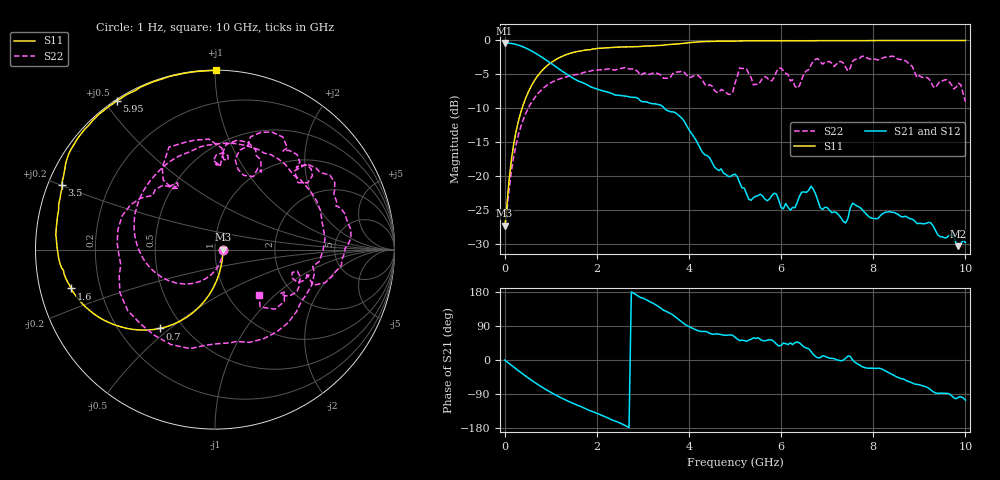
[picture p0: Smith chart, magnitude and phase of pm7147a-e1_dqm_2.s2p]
# GHz S DB R 50
! S-Parameters data
! Freq  dbS11  angS11  dbS21  angS21  dbS12  angS12  dbS22  angS22
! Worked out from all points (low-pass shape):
!   279 points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, 1 Hz to 10 GHz, reference 50 ohm
!   highest |S21| = -0.38 dB at 2 Hz (marker M1); lowest = -30.3 dB at 9.85 GHz (marker M2)
!   |S21| within 3 dB of the highest: start of sweep to 1.004 GHz
!   lowest |S11| = -27.3 dB at 1.6 Hz (marker M3), VSWR 1.09, Z = 54.5 - j1.04e-07 ohm
!   |S11| at or under -10 dB: start of sweep to 380.1 MHz
!   |S22| runs from -27.3 to -2.3 dB; largest |S21 - S12| = 0
!   S11 on the Smith chart (normalised r, x): 1 Hz: 1.09, -0.00; 700 MHz: 0.37, -0.46; 1.6 GHz: 0.09, -0.13; 3.5 GHz: 0.04, +0.20; 5.95 GHz: 0.00, +0.54; 10 GHz: 0.00, +1.01
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1e-09  -27.30 -0.0  -0.38 -0.0  -0.38 -0.0  -27.30 -0.0
1.6e-09  -27.30 -0.0  -0.38 -0.0  -0.38 -0.0  -27.30 -0.0
2e-09  -27.30 -0.0  -0.38 -0.0  -0.38 -0.0  -27.30 -0.0
0.25  -13.38 -92.7  -0.61 -23.6  -0.61 -23.6  -15.33 -108.1
0.7  -5.40 -125.1  -2.02 -62.9  -2.02 -62.9  -8.03 -170.7
1.6  -1.61 -164.9  -6.01 -120.1  -6.01 -120.1  -5.01 105.0
1.7  -1.49 -167.9  -6.25 -125.4  -6.25 -125.4  -4.75 98.0
2.65  -0.96 169.9  -8.24 -175.0  -8.24 -175.0  -4.06 20.4
3.35  -0.75 158.9  -9.48 140.2  -9.48 140.2  -4.95 -61.2
3.5  -0.66 157.1  -10.25 129.0  -10.25 129.0  -5.58 -80.7
3.9  -0.43 151.4  -11.95 95.3  -11.95 95.3  -4.70 -155.6
4.3  -0.20 145.0  -16.55 75.3  -16.55 75.3  -5.96 145.3
5.05  -0.10 134.4  -20.10 55.3  -20.10 55.3  -5.31 122.7
5.3  -0.06 131.1  -23.42 52.6  -23.42 52.6  -4.93 86.1
5.95  -0.06 123.5  -23.58 37.2  -23.58 37.2  -4.12 78.5
6.3  -0.05 119.7  -24.67 45.5  -24.67 45.5  -6.75 62.2
6.7  -0.06 115.9  -21.94 14.3  -21.94 14.3  -3.06 68.5
7.4  -0.04 109.2  -26.92 4.5  -26.92 4.5  -3.92 35.8
8.35  -0.03 101.3  -25.24 -34.4  -25.24 -34.4  -2.42 11.0
8.85  -0.02 97.5  -26.36 -60.6  -26.36 -60.6  -3.87 -16.8
9.85  -0.02 90.6  -30.33 -98.0  -30.33 -98.0  -6.32 -36.8
10  -0.02 89.6  -29.81 -106.0  -29.81 -106.0  -9.01 -45.9
